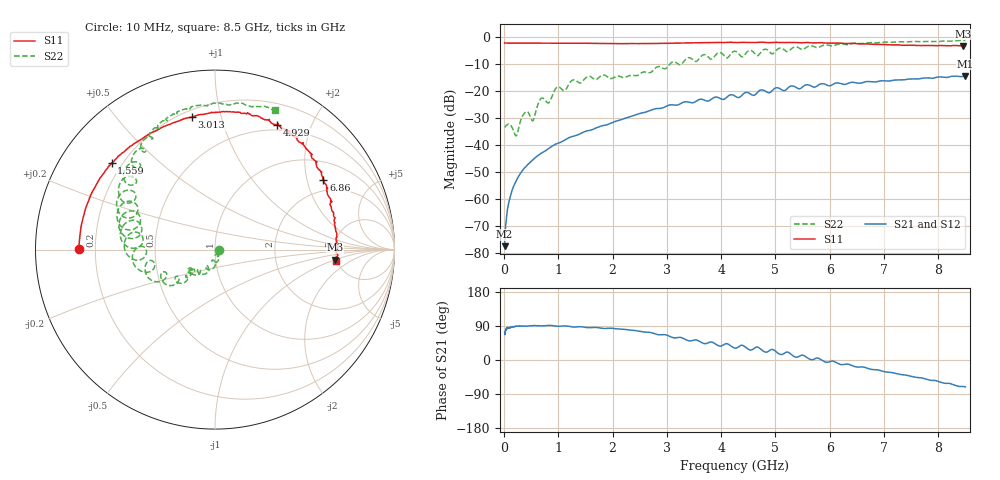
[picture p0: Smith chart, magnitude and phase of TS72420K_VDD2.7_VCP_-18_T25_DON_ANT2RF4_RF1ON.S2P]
!Agilent Technologies,E5071C,MY46417908,A.11.23
!Date: Thu Oct 03 16:40:47 2019
!Data & Calibration Information:
!Freq	S11:SOLT2(ON)	S21:SOLT2(ON)	S12:SOLT2(ON)	S22:SOLT2(ON)
!PortZ  Port1:50+j0  Port2:50+j0
!Above PortZ is port z conversion or system Z0 setting when saving the data.
!When reading, reference impedance value at option line is always used.
# Hz S dB R 50
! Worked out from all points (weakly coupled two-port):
!   1601 points, 10 MHz to 8.5 GHz, reference 50 ohm
!   highest |S21| = -14.58 dB at 8.5 GHz (marker M1); lowest = -77.5 dB at 10 MHz (marker M2)
!   lowest |S11| = -3.5 dB at 8.458 GHz (marker M3), VSWR 5.09, Z = 244 - j50.1 ohm
!   |S11| at or under -10 dB: nowhere
!   |S22| runs from -36.7 to -1.4 dB; largest |S21 - S12| = 0.0021
!   S11 on the Smith chart (normalised r, x): 10 MHz: 0.14, +0.00; 1.559 GHz: 0.16, +0.35; 3.013 GHz: 0.24, +0.81; 4.929 GHz: 0.43, +1.52; 6.86 GHz: 1.59, +2.53; 8.5 GHz: 4.88, -1.13
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1e7  -2.38 179.8  -77.46 73.6  -78.76 75.4  -33.61 -0.2
6.836875e7  -2.40 178.1  -63.36 84.8  -63.25 83.9  -32.44 -19.6
1.16125e8  -2.41 176.7  -58.90 86.4  -59.05 86.2  -32.65 -38.8
2.2225e8  -2.42 173.6  -53.41 89.4  -53.42 89.0  -36.74 -46.9
3.28375e8  -2.42 170.7  -49.78 89.5  -49.74 89.4  -29.78 -38.4
4.13275e8  -2.42 168.5  -47.82 89.5  -47.83 89.5  -27.71 -75.5
5.300125e8  -2.44 165.3  -45.60 90.7  -45.59 90.3  -31.16 -78.0
6.67975e8  -2.42 162.0  -43.33 90.0  -43.31 90.1  -23.16 -81.0
8.271625e8  -2.44 157.6  -41.34 91.4  -41.34 91.2  -24.45 -97.4
9.757375e8  -2.44 154.2  -39.58 89.1  -39.56 89.0  -18.70 -104.8
1.426769e9  -2.49 142.9  -35.64 87.5  -35.63 87.7  -16.94 -125.0
1.559425e9  -2.49 140.1  -34.75 85.2  -34.73 85.2  -14.66 -132.8
2.222706e9  -2.62 122.0  -30.27 80.8  -30.26 80.9  -15.15 -138.7
2.843538e9  -2.54 104.4  -26.59 66.7  -26.58 66.7  -11.09 -140.2
3.013338e9  -2.51 99.9  -25.52 64.9  -25.51 64.9  -11.17 -138.8
4.255e9  -2.17 75.4  -21.99 31.4  -21.98 31.3  -5.44 168.8
4.928894e9  -2.20 63.7  -20.20 27.9  -20.17 27.5  -6.31 152.6
5.671769e9  -2.34 53.2  -18.41 0.8  -18.33 1.1  -3.45 134.1
6.860369e9  -2.89 32.6  -16.73 -25.7  -16.70 -25.6  -2.32 110.3
7.088538e9  -3.04 27.8  -16.42 -32.5  -16.40 -31.9  -2.10 106.3
8.45755e9  -3.46 -4.8  -14.73 -69.8  -14.78 -70.3  -1.48 68.4
8.5e9  -3.41 -5.4  -14.58 -70.9  -14.61 -71.3  -1.44 66.9
